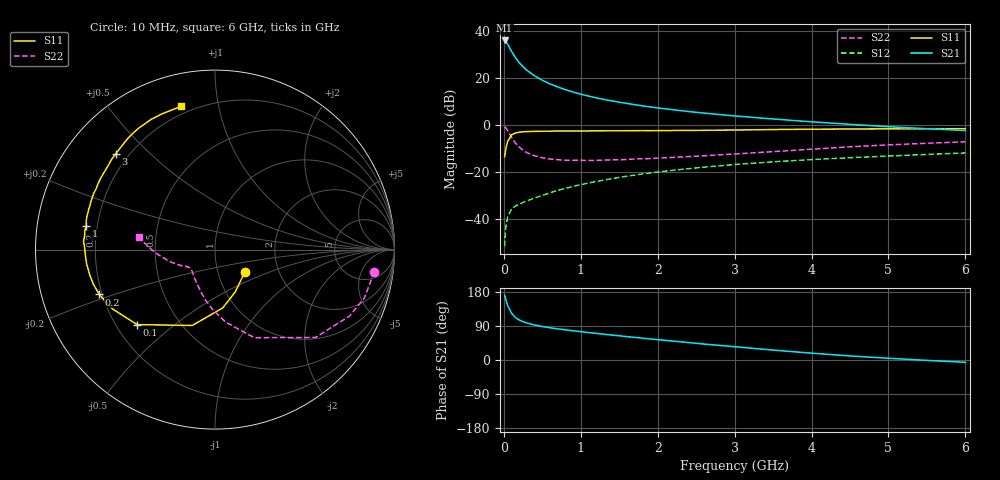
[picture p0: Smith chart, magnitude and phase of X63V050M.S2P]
! SIEMENS Small Signal Semiconductors
! BFP193W
! Si NPN RF Bipolar Junction Transistor in SOT343
! VCE = 3 V  IC = 50 mA
! Common Emitter S-Parameters:  April 1994
# GHz  S  MA  R  50
!  f  S11  S21  S12  S22
! GHz  MAG  ANG  MAG  ANG  MAG  ANG  MAG  ANG
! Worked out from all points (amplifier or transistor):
!   40 points, 10 MHz to 6 GHz, reference 50 ohm
!   highest |S21| = 35.8 dB at 10 MHz (marker M1)
!   |S21| within 3 dB of that: start of sweep to 72.8 MHz
!   unconditionally stable (mu >= 1): 574.1 MHz to 3.92 GHz
!   at 200 MHz: K = 0.59, MSG = 30.1 dB, |S12| = -33.9 dB
!   at 1.5 GHz: K = 1.14, MAG = 13.8 dB, |S12| = -22.4 dB
!   at 6 GHz: K = 0.94, MSG = 4.8 dB, |S12| = -12.0 dB
!   S11 on the Smith chart (normalised r, x): 10 MHz: 1.35, -0.35; 100 MHz: 0.29, -0.37; 200 MHz: 0.19, -0.18; 1 GHz: 0.16, +0.09; 3 GHz: 0.15, +0.39; 6 GHz: 0.16, +0.78
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0.01  0.2079 -36.7  61.72 171.0  0.0026 80.6  0.8963 -8.0
0.02  0.262 -64.6  60.17 163.8  0.0053 74.6  0.875 -17.9
0.03  0.328 -82.5  57.78 156.5  0.0072 72.0  0.836 -26.3
0.05  0.4413 -106.7  51.11 143.8  0.011 62.2  0.7437 -41.2
0.1  0.6027 -136.1  36.23 123.5  0.016 48.9  0.5372 -66.0
0.15  0.6624 -150.4  26.73 112.2  0.0186 45.1  0.4085 -81.6
0.2  0.6914 -158.8  20.84 105.6  0.0202 45.8  0.3327 -92.5
0.25  0.7042 -164.0  17.07 100.9  0.0222 47.3  0.2866 -100.6
0.3  0.7113 -168.0  14.33 97.5  0.024 48.7  0.2527 -107.3
0.4  0.72 -173.8  10.89 92.3  0.0273 52.7  0.2171 -117.1
0.5  0.7232 -177.7  8.782 88.3  0.0313 55.4  0.1979 -124.5
0.6  0.727 178.9  7.333 85.0  0.0355 57.5  0.186 -130.1
0.7  0.7341 176.3  6.347 82.3  0.0397 59.5  0.179 -134.1
1  0.7301 169.6  4.439 74.8  0.0528 62.4  0.1743 -141.9
1.1  0.7343 167.6  4.063 72.5  0.0574 62.5  0.1731 -143.5
1.6  0.742 158.4  2.821 61.6  0.08 62.3  0.1811 -148.2
2.2  0.7506 148.5  2.073 49.8  0.107 59.4  0.2009 -153.6
3  0.7682 136.1  1.533 35.1  0.1416 53.7  0.2369 -161.1
3.2  0.7739 133.0  1.444 31.5  0.1496 52.1  0.2489 -163.0
4.5  0.8084 116.0  1.015 10.7  0.1979 42.3  0.3378 -177.6
5.5  0.814 107.5  0.818 -1.0  0.2323 35.4  0.4018 173.9
6  0.82 103.3  0.751 -6.1  0.2501 32.5  0.4317 170.7
